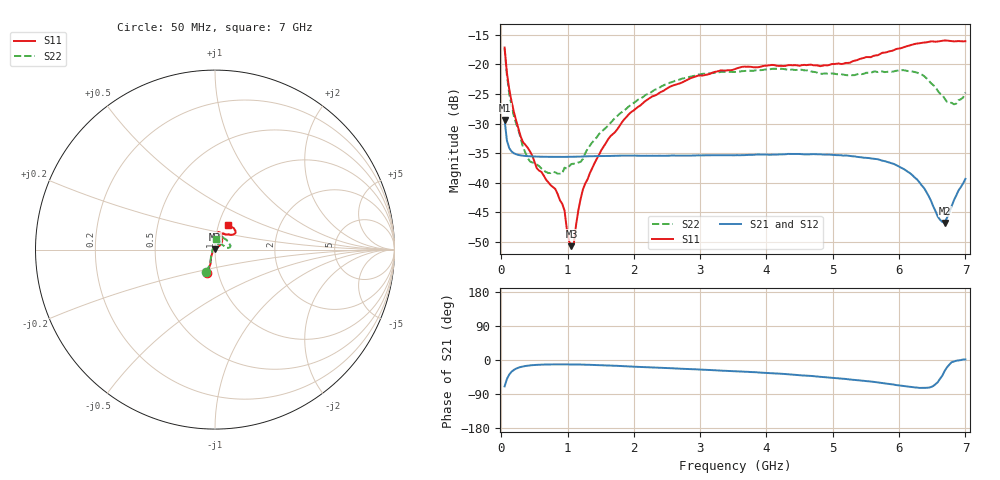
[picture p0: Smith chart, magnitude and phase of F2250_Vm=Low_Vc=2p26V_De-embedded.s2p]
! Integrated Device Technology
! Corporate Headquarters
! 6024 Silver Creek Valley Road
! San Jose, CA 95138  USA
! Phone:  1-408-284-8200
! Toll Free:  1-800-223-1366
! Webpage:  http://www.idt.com/
! Timing and RF Division
! 515 Groton Road, Suite 102
! Westford, MA 01886-6024
! Device:  F2250
! Description: Voltage Variable RF Attenuator
! Frequency:  50.0 -  6000.00 MHz
! Package:  3x3 mm Thin QFN Plastic Package: 16 pin
! Ports:  2 RF, 3 DC
!  Pin  1  = GND
!  Pin  2  = NC
!  Pin  3  = RF1  = Port 1
!  Pin  4  = NC
!  Pin  5  = GND
!  Pin  6  = GND
!  Pin  7  = GND
!  Pin  8  = GND
!  Pin  9  = NC
!  Pin 10  = RF2  = Port 2
!  Pin 11  = NC
!  Pin 12  = GND
!  Pin 13  = GND
!  Pin 14  = VCNTRL
!  Pin 15  = VDD
!  Pin 16  = VMODE
! Vcntrl:  2.260 Volts
! Vmode:  +0.000 Volts
! Vdd:  +3.30  Volts
! Current:  1.177 mA
! Data:  The device was measured on a the F2250 evaluation board which has
!  individual transmission lines to the RF pins.  Data was collected
!  using a calibrated network analyzer.  The evaluation board was
!  de-embedded using a TRL calibration technique.
!  The reference plane is the edge of the package pin.
! Misc:  SN 10
!  Action Tracker AT0258
! Date Measured:  2014-11-26
! Date:  2015-10-15  MJV
! Note:
!  Integrated Device Technology supplies this data as a sample of measured
!  data at the package pin for this product.  Your particular data for this
!  product may vary.
!  Data was taken at 25 degrees C.
!  Integrated Device Technology reserves the right to change this data at anytime.
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# GHz S dB R 50
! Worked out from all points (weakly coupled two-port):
!   201 points, 50 MHz to 7 GHz, reference 50 ohm
!   highest |S21| = -29.39 dB at 50 MHz (marker M1); lowest = -46.8 dB at 6.687 GHz (marker M2)
!   lowest |S11| = -50.7 dB at 1.058 GHz (marker M3), VSWR 1.01, Z = 49.8 + j0.244 ohm
!   |S11| at or under -10 dB: start of sweep to end of sweep
!   |S22| runs from -38.5 to -17.3 dB; largest |S21 - S12| = 6e-05
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0.05  -17.18 -108.6  -29.39 -69.6  -29.39 -69.6  -17.35 -110.7
0.08475  -21.45 -107.5  -32.88 -50.2  -32.88 -50.2  -21.85 -109.4
0.15425  -26.23 -116.6  -34.71 -31.0  -34.71 -31.0  -27.02 -120.9
0.29325  -32.22 -127.8  -35.38 -18.4  -35.38 -18.4  -32.51 -135.0
0.3975  -34.08 -141.8  -35.51 -15.0  -35.50 -15.0  -35.79 -158.5
0.6755  -39.47 -163.7  -35.62 -11.9  -35.61 -11.9  -38.17 158.4
0.91875  -43.54 157.8  -35.63 -11.5  -35.63 -11.5  -38.43 129.3
0.9535  -44.67 170.2  -35.63 -11.6  -35.63 -11.6  -37.44 127.5
1.023  -49.88 143.8  -35.62 -11.6  -35.62 -11.6  -37.23 111.0
1.05775  -50.69 122.9  -35.61 -11.6  -35.62 -11.7  -36.83 105.8
1.0925  -50.42 89.5  -35.61 -11.7  -35.61 -11.7  -36.77 101.1
1.162  -44.66 56.9  -35.59 -11.9  -35.58 -11.9  -36.57 90.0
1.2315  -41.10 44.4  -35.55 -12.1  -35.56 -12.1  -35.96 80.5
1.6485  -32.11 41.9  -35.47 -14.7  -35.47 -14.7  -29.88 61.9
2.37825  -24.87 47.4  -35.43 -20.3  -35.43 -20.4  -24.02 55.5
3.525  -20.80 72.5  -35.36 -29.6  -35.36 -29.7  -21.30 74.1
4.7065  -20.17 72.4  -35.16 -42.7  -35.16 -42.7  -21.28 71.9
5.85325  -17.82 40.5  -36.59 -63.4  -36.59 -63.4  -21.21 22.2
6.27025  -16.50 40.1  -39.43 -72.7  -39.43 -72.7  -21.42 8.9
6.68725  -15.99 48.8  -46.77 -28.7  -46.72 -28.2  -25.79 27.8
6.861  -16.12 55.1  -42.16 -2.0  -42.12 -2.0  -26.65 57.9
7  -16.12 63.2  -39.34 1.3  -39.30 1.2  -24.76 83.5
